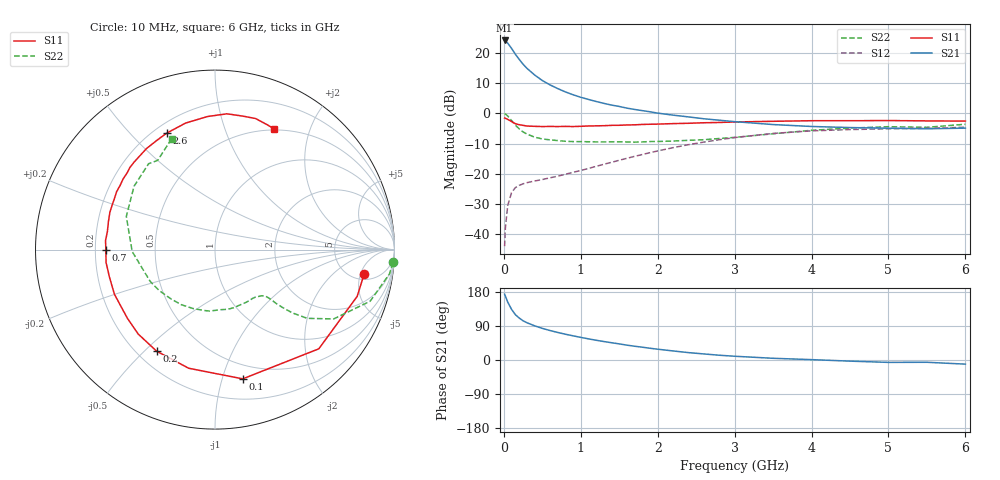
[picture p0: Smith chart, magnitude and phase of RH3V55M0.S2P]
! SIEMENS Small Signal Semiconductors
! BFR106
! Si NPN RF Bipolar Junction Transistor in SOT23
! VCE = 3.5 V  IC = 5 mA
! Common Emitter S-Parameters:  August  1996
# GHz  S  MA  R  50
!  f  S11  S21  S12  S22
! GHz  MAG  ANG  MAG  ANG  MAG  ANG  MAG  ANG
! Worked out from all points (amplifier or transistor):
!   36 points, 10 MHz to 6 GHz, reference 50 ohm
!   highest |S21| = 24.1 dB at 10 MHz (marker M1)
!   |S21| within 3 dB of that: start of sweep to 110.1 MHz
!   unconditionally stable (mu >= 1): 626.9 MHz to 2.017 GHz; 4.62 GHz to end of sweep
!   at 250 MHz: K = 0.50, MSG = 19.8 dB, |S12| = -23.3 dB
!   at 1.4 GHz: K = 1.14, MAG = 7.2 dB, |S12| = -16.1 dB
!   at 6 GHz: K = 1.02, MAG = -1.1 dB, |S12| = -4.5 dB
!   S11 on the Smith chart (normalised r, x): 10 MHz: 6.31, -5.80; 100 MHz: 0.37, -1.17; 200 MHz: 0.28, -0.54; 700 MHz: 0.24, -0.00; 2.6 GHz: 0.25, +0.64; 6 GHz: 0.49, +1.49
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0.01  0.8426 -9.1  16.12 173.6  0.0064 87.4  0.9935 -4.1
0.02  0.8339 -18.2  15.91 168.7  0.0128 79.4  0.9817 -7.9
0.05  0.8 -43.7  14.58 152.9  0.0299 68.5  0.9111 -18.4
0.1  0.7365 -77.9  11.94 133.8  0.0491 53.8  0.7657 -30.3
0.15  0.6771 -102.5  9.541 119.6  0.0595 44.9  0.6408 -36.7
0.2  0.6527 -119.9  7.842 110.7  0.0648 40.9  0.5566 -39.3
0.25  0.6359 -132.3  6.522 103.5  0.0687 38.6  0.495 -40.6
0.3  0.6202 -141.9  5.584 98.4  0.0718 38.1  0.4576 -41.3
0.4  0.6131 -156.0  4.334 90.2  0.0765 38.7  0.4059 -41.9
0.5  0.6076 -165.3  3.509 83.5  0.0809 40.9  0.3793 -42.8
0.6  0.6111 -173.2  2.972 77.8  0.0864 43.3  0.3664 -44.6
0.7  0.608 -179.8  2.581 72.7  0.0919 46.6  0.3564 -47.1
0.9  0.6079 170.5  2.039 63.8  0.1066 51.9  0.343 -52.4
1.1  0.6214 160.6  1.707 55.8  0.1234 56.3  0.3409 -59.7
1.6  0.6459 142.5  1.226 39.2  0.1816 61.2  0.3382 -80.4
2.2  0.6802 124.1  0.939 23.9  0.2723 58.0  0.3502 -110.1
2.6  0.7025 112.6  0.818 16.0  0.3366 52.5  0.3685 -132.1
3.5  0.7427 93.2  0.656 4.5  0.4682 35.8  0.4616 -178.7
4.5  0.7596 78.3  0.585 -3.0  0.5422 16.5  0.5726 142.0
5  0.7645 72.8  0.571 -6.3  0.5584 8.6  0.6049 127.7
5.5  0.754 67.3  0.559 -6.0  0.5669 4.7  0.5909 122.7
6  0.7486 63.9  0.572 -10.9  0.5938 -3.1  0.6639 111.3
